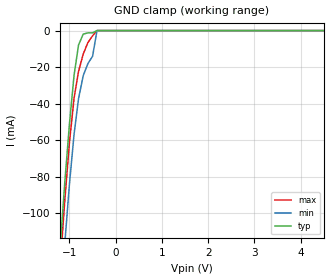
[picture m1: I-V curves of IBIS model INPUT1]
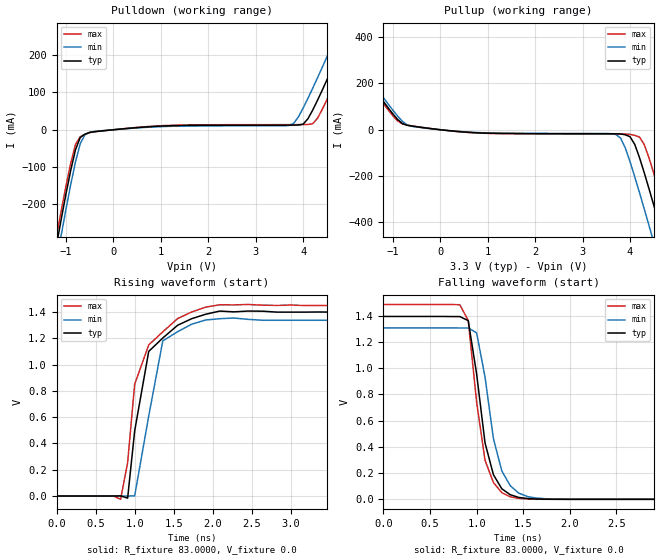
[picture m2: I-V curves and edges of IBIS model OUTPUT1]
|   PERICOM SEMICONDUCTOR CORP
|   IBIS Model of PI6C557-03A
|   Product Family: 6C
|   16 Pin TSSOP Package
[IBIS Ver] 3.2
[Comment char] |_char
[File Name] pi6c557-03a.ibs
[File Rev] 2.1
[Source] File originated at Pericom Semiconductor Corp.
[Date] 07/30/2011
[Disclaimer] (C) Copyright PERICOM Semiconductor Corporation
   All rights reserved
  Pericom Semiconductor Corporation hereby grants the user of
  this IBIS model a non-exclusive, nontransferable license to
  use this IBIS model under the following terms.
  This IBIS model is provided on an "AS IS" basis and Pericom
  makes absolutely no warranty with respect to the information
  contained herein. PERICOM DISCLAIMS AND CUSTOMER WAIVES ALL
  WARRANTIES, EXPRESSED OR IMPLIED, INCLUDING WARRANTIES OF
  MERCHANTABILITY OR FITNESS FOR A PARTICULAR PURPOSE. The
  entire risk as to quality and performance is with the customer.
  Accordingly, in no event shall the company be liable for any
  damages, whether in contract or tort, including any lost
  profits or other incidental, consequential, exemplary, or
  punitive damages arising out of the use or application of the
  IBIS model provided in this package. Further, Pericom reserves
  the right to make changes without notice to any product herein
  to improve reliability, function, or design. Pericom does not
  convey any license under patent rights or any other intellectual
  property rights, including those of third parties.
  The user is granted this license only to use the IBIS model
  and is not granted rights to sell, load, rent, lease or license
  the IBIS model in whole or in part, or in modified form to anyone
  other than user. User may modify the IBIS model to suit its specific
  application but rights to derivative works and such modifications
  shall belong to Pericom.
  Pericom is not obligated to provide maintenance or support
  for the licensed IBIS model.
  Contact Pericom at ATTN: APPLICATION ENGINEERING / IBIS MODELS
  3545 North First Street, San Jose, CA 95134
[Component] PI6C557-03A
[Manufacturer] Pericom Semiconductor Corp.
[Package]
|   typ   min   max
R_pkg   3.400e-02   2.800e-02   3.900e-02
L_pkg   3.404e-09   2.704e-09   4.545e-09
C_pkg   4.280e-13   2.990e-13   5.710e-13
[Pin]   signal_name   model_name   R_pin   L_pin   C_pin
1   S0   INPUT1   3.800e-02   4.545e-09   5.640e-13
2   S1   INPUT1   3.900e-02   4.133e-09   5.710e-13
3   SS0   INPUT1   3.500e-02   3.598e-09   4.890e-13
4   X1   INPUT1   2.800e-02   3.087e-09   4.080e-13
| 5   X2   OUTPUT   3.200e-02   2.990e-09   3.490e-13
6   OE   INPUT1   3.200e-02   2.774e-09   3.180e-13
7   GNDX   POWER   3.800e-02   4.545e-09   5.640e-13
8   SS1   INPUT1   3.100e-02   2.704e-09   2.990e-13
| 9   IREF   OUTPUT   3.200e-02   2.774e-09   3.180e-13
10   /CLK1   OUTPUT1   3.200e-02   2.990e-09   3.490e-13
11   CLK1   OUTPUT1   2.800e-02   3.087e-09   4.080e-13
12   VDDA   POWER   3.500e-02   3.598e-09   4.890e-13
13   GNDA   POWER   3.900e-02   4.133e-09   5.710e-13
14   /CLK0   OUTPUT1   3.200e-02   2.990e-09   3.490e-13
15   CLK0   OUTPUT1   3.200e-02   2.990e-09   3.490e-13
16   VDDX   POWER   3.900e-02   4.133e-09   5.710e-13
[Diff Pin] inv_pin  vdiff   tdelay_typ  tdelay_min   tdelay_max
11   10   NA   0ns   -0.05ns   0.05ns
15   14   NA   0ns   -0.05ns   0.05ns
| Models and submodels in the file (2): INPUT1 (Input), OUTPUT1 (Output)
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|   Model INPUT1
[Model] INPUT1
Model_type Input
Vinl = 0.80V
Vinh = 2.00V
| variable   typ   min   max
C_comp   4.00pF   3.8pF   4.2pF
[Voltage Range]   3.30V   3.135V   3.465V
[GND Clamp Reference]   0.00V   0.00V   0.00V
[POWER Clamp Reference]  3.30V   3.135V   3.465V
[temperature range]   25   70   0
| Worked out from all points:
|   GND clamp passes 1 mA (typ) near -0.48 V on its own axis
[GND Clamp]
| Voltage   I(typ)   I(min)   I(max)
-3.3V     -916.6mA   -1.057A    -1.075A
-1.202V   -119.6mA   -152.7mA   -129.7mA
-1.101V   -83.43mA   -117.1mA   -93.38mA
-999.5mV  -51.29mA   -84.23mA   -61.35mA
-898.4mV  -24.31mA   -56.66mA   -36.88mA
-802.3mV  -7.88mA    -37.26mA   -22.34mA
-701.1mV  -1.92mA    -24.67mA   -12.83mA
-599.9mV  -1.27mA    -18.1mA    -6.55mA
-498.7mV  -1.22mA    -14.03mA   -2.87mA
-403mV    0A         0A         0A
6.602V    0A         0A         0A
[POWER Clamp]   |Note: Vtable = Vcc - Voutput
| Voltage   I(typ)   I(min)   I(max)
-3.3V     0A         0A         0A
0V        0A         0A         0A
|   Model OUTPUT1
[Model]  OUTPUT1
Model_type Output
C_comp   5.5000pF   5.0000pF   6.0000pF
Vref = 0.00V
Vmeas = 0.35V
[Temperature Range]   25.0000   70.0000   0.0
[Voltage Range]   3.3000V   3.1350V   3.4650V
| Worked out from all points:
|   slope of the pulldown table from 0 to 0.495 V, typ, clamps not added: 87.5 ohm
|   slope of the pullup table from 0 to 0.495 V, typ, clamps not added: 51.4 ohm
|   rising waveform, R_fixture 83.0000, V_fixture 0.0: 20-80 % time 247ps typ, 246ps min, 280ps max; typ from 0 V to 1.4 V
|   falling waveform, R_fixture 83.0000, V_fixture 0.0: 20-80 % time 182ps typ, 194ps min, 155ps max; typ from 1.39 V to 0 V
[Pulldown]
|Voltage   I(typ)   I(min)   I(max)
-3.3V     -1.864A    -1.903A    -1.842A
-1.2V     -309mA     -351.5mA   -285.8mA
-1.1V     -239mA     -281.1mA   -216.3mA
-800mV    -53.54mA   -86.05mA   -39.29mA
-700mV    -20.77mA   -37.28mA   -18.67mA
-500mV    -7.206mA   -6.909mA   -7.537mA
3.7V      12.34mA    11.24mA    13.71mA
4.2V      52.37mA    110.9mA    16.14mA
4.8V      218.8mA    281mA      164mA
5V        276.8mA    339.2mA    221.7mA
5.2V      335.4mA    397.7mA    280.1mA
6.6V      753.8mA    814.8mA    699mA
[Pullup]
|Voltage   I(typ)   I(min)   I(max)
-3.3V     730.8mA    746.6mA    722.2mA
-2.3V     437.8mA    454mA      428.8mA
-800mV    26.77mA    36.48mA    25.04mA
600mV     -11.15mA   -10.19mA   -11.93mA
3.7V      -17.37mA   -20.36mA   -18.45mA
4V        -30.01mA   -138mA     -19.92mA
4.2V      -120.7mA   -272mA     -31.84mA
4.4V      -254.8mA   -413.4mA   -121.8mA
4.5V      -325.2mA   -485.3mA   -187.7mA
4.7V      -469.1mA   -630.7mA   -327.8mA
4.9V      -615.2mA   -777.4mA   -472.4mA
6.6V      -1.881A    -2.043A    -1.737A
[Ramp]
| variable   typ   min   max
dV/dt_r  0.5146/77.3507p   0.4826/84.7389p   0.5491/78.8107p
dV/dt_f  0.3648/0.4177n   0.3144/0.4513n   0.4056/0.3997n
R_load = 50.0000
[Rising Waveform]
R_fixture= 83.0000
V_fixture= 0.0
|time   V(typ)   V(min)   V(max)
0s        0V         0V         0V
820ps     1.505mV    -7.234uV   -25.08mV
910ps     -16.18mV   17.71uV    254.3mV
1ns       495.1mV    1.217mV    851mV
1.18ns    1.101V     608.8mV    1.15V
1.36ns    1.203V     1.181V     1.25V
1.55ns    1.3V       1.251V     1.351V
1.91ns    1.384V     1.34V      1.438V
2.09ns    1.408V     1.35V      1.456V
9ns       1.397V     1.338V     1.448V
[Falling Waveform]
R_fixture= 83.0000
V_fixture= 0.0
|time   V(typ)   V(min)   V(max)
0s        1.393V     1.306V     1.484V
820ps     1.392V     1.305V     1.482V
910ps     1.361V     1.305V     1.362V
1ns       954.9mV    1.268V     740.7mV
1.09ns    430.4mV    932mV      297.7mV
1.18ns    187.5mV    462.6mV    127.9mV
1.27ns    80.44mV    216.6mV    50.82mV
1.36ns    35.1mV     104mV      19.3mV
1.82ns    291.5uV    1.489mV    -32.66uV
9ns       0V         0V         0V
